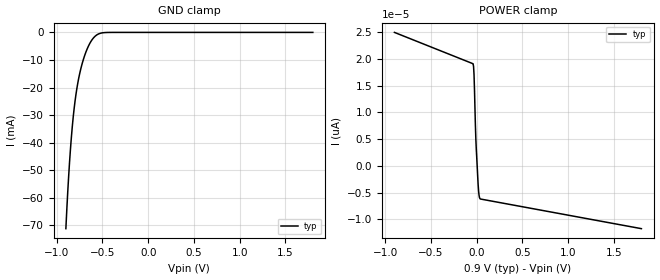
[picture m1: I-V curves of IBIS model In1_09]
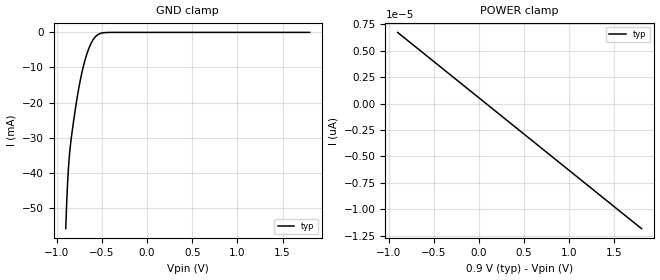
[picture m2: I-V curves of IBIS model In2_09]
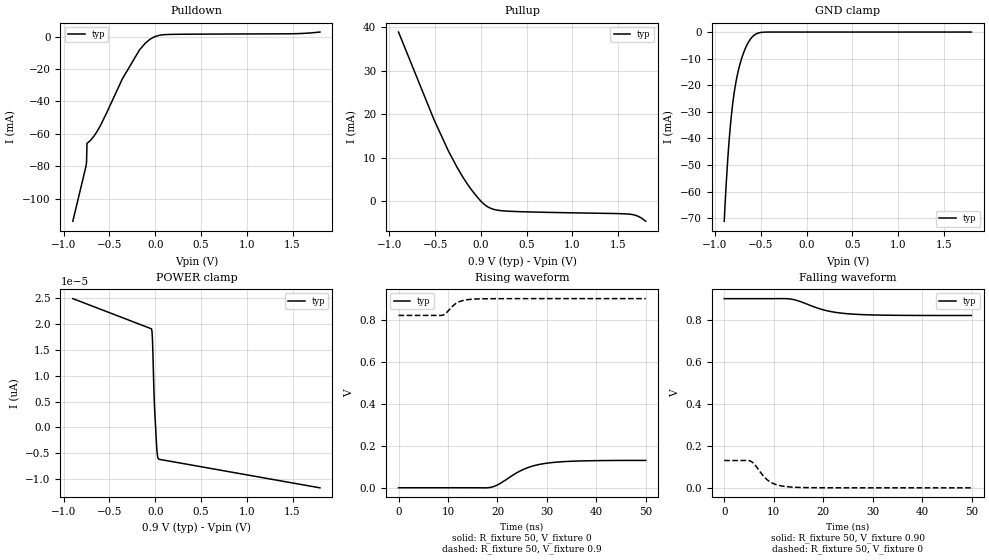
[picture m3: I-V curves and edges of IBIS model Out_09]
|//////////////////////////////////////////////////////////////////////////////
|//////////////////////////////////////////////////////////////////////////////
|   @@@@@@@   @@@@@@@   @@@@@@@   @@@@@@@   @@@@@@@   @@@@@@   @@
|   @@@@@@@@@   @@@@@@@@@   @@@@@@@@@   @@@@@@@@@   @@@@@@@@@ @@@@@@@@  @
|   @@@   @@@ @@@   @@@ @@@   @@@   @@@ @@@   @@@@   @@@  @
|   @@   @@ @@   @@ @@@@@@@@@@@ @@@@@@@@@@@ @@   @@   @@ @@
|   @@@   @@@ @@   @@   @@@ @@@   @@   @@   @@ @@
|   @@@@@@@@@  @@   @@  @@@@@@@@@   @@@@@@@@@  @@   @@   @@ @@
|   @@@@@@@   @@   @@   @@@@@@@   @@@@@@@   @@   @@   @@ @@
|   IBIS Model of NL3V2T244
|   2-Bit Dual-Supply Level Translator
|   Package Type: UDFN8, CASE 517AJ
|   Micro8, CASE 846A-02
|   The model is covering the following Vccs:
|   0.9V, 1.2V, 1.5V, 1.8V, 2.5V, 3.3V
|//////////////////////////////////////////////////////////////////////////////
|//////////////////////////////////////////////////////////////////////////////
[IBIS Ver]   3.2
|   7.2 compatible
|//////////////////////////////////////////////////////////////////////////////
[Comment Char] |_char
|//////////////////////////////////////////////////////////////////////////////
[File Name]   nl3v2t244_va_r0.ibs
|//////////////////////////////////////////////////////////////////////////////
[File Rev]   0.0
|   0.0 - Feb 19, 2025 - File created
|//////////////////////////////////////////////////////////////////////////////
[Date]   February 19, 2025
|//////////////////////////////////////////////////////////////////////////////
[Source]   From lab measurements and simulations at onsemi
|//////////////////////////////////////////////////////////////////////////////
[Notes]   - The currents greater than +/- 100 mA are extrapolated
|//////////////////////////////////////////////////////////////////////////////
[Disclaimer]
   - onsemi Corporation hereby grants
   the user of this IBIS model a license to use this model
   under the following terms. This license is nonexclusive
   and nontransferable. Before using this IBIS model.
   After reading the terms and conditions of this license,
   the user either must accept these terms,
   or the IBIS model should be returned to onsemi within 30 days.
   - The user is hereby granted a license to use the IBIS model.
   This shall not be construed as a right to sell,
   or otherwise profit either by leasing or renting this software.
   - The user may modify the IBIS model to suit his specific
   applications but rights to derivative works and such
   modifications shall belong to onsemi.
   - This IBIS model is provided on an "as is" basis.
   onsemi makes absolutely no warranty with respect
   to the information contained herein.
   By use of this IBIS model, the user assumes full risk as to the
   quality and suitablility of the model to his particular use,
   and by using this model assumes the entire risk.
   Under all circumstances the user shall not hold
   onsemi liable in any way for the results obtained.
   onsemi reserves the right to make to improve
   the model for reliability, function, or design.
   onsemi does not convey any license under patent
   rights or any other intellectual property rights,
   including those of third parties.
   - onsemi is not obligated to provide maintenance
   or support for the licensed IBIS model.
   - Cont onsemi at ATTN:LOGIC APPLICATIONS/IBIS MODEL.
   5701 N Pima Rd, Scottsdale, AZ 85250
|//////////////////////////////////////////////////////////////////////////////
[Copyright]   (c) 2025 onsemi Corp.
|//////////////////////////////////////////////////////////////////////////////
|//////////////////////////////////////////////////////////////////////////////
[Component]   NL3V2T244DMR2G
|//////////////////////////////////////////////////////////////////////////////
[Manufacturer]  onsemi
|   Data Sheet: NL3V2T244/D, Rev. P1,  October, 2024
|//////////////////////////////////////////////////////////////////////////////
[Package]
|   Micro8
| CASE 846A-02
|  DM SUFFIX
| variable   typ   min   max
R_pkg   0.1829   0.0061   0.2446
L_pkg   2.8385nH   1.565nH   3.89485nH
C_pkg   0.4567pF   0.38386pF   0.53234pF
|//////////////////////////////////////////////////////////////////////////////
[Pin] signal_name   model_name   R_pin   L_pin   C_pin
1   VCCA   POWER   0.1862   2.8664nH   0.4560pF
2   A1   In1   0.2446   3.8949nH   0.5323pF
3   A2   In1   0.2357   3.2912nH   0.4714pF
4   OE   In2   0.1867   2.8664nH   0.4559pF
5   GND   GND   0.1866   1.5684nH   0.3839pF
6   B2   Out   0.2341   3.8112nH   0.5277pF
7   B1   Out   0.0061   1.5650nH   0.3853pF
8   VCCB   POWER   0.1830   2.8445nH   0.4412pF
|//////////////////////////////////////////////////////////////////////////////
|//////////////////////////////////////////////////////////////////////////////
[Component]   NL3V2T244DMR2G-Q
|//////////////////////////////////////////////////////////////////////////////
[Manufacturer]  onsemi
|   Data Sheet: NL3V2T244/D, Rev. P1,  October, 2024
|//////////////////////////////////////////////////////////////////////////////
[Package]
R_pkg   0.1829   0.0061   0.2446
L_pkg   2.8385nH   1.565nH   3.89485nH
C_pkg   0.4567pF   0.38386pF   0.53234pF
|//////////////////////////////////////////////////////////////////////////////
[Pin] signal_name   model_name   R_pin   L_pin   C_pin
1   VCCA   POWER   0.1862   2.8664nH   0.4560pF
2   A1   In1   0.2446   3.8949nH   0.5323pF
3   A2   In1   0.2357   3.2912nH   0.4714pF
4   OE   In2   0.1867   2.8664nH   0.4559pF
5   GND   GND   0.1866   1.5684nH   0.3839pF
6   B2   Out   0.2341   3.8112nH   0.5277pF
7   B1   Out   0.0061   1.5650nH   0.3853pF
8   VCCB   POWER   0.1830   2.8445nH   0.4412pF
|//////////////////////////////////////////////////////////////////////////////
|//////////////////////////////////////////////////////////////////////////////
[Component]   NL3V2T244MUTAG
|//////////////////////////////////////////////////////////////////////////////
[Manufacturer]  onsemi
|   Data Sheet: NL3V2T244/D, Rev. P1,  October, 2024
|//////////////////////////////////////////////////////////////////////////////
[Package]
|   UDFN_8
| CASE 517AJ
|  MU SUFFIX
| variable   typ   min   max
R_pkg   0.0451   0.0011   0.0571
L_pkg   0.3714nH   0.01454nH  0.4787nH
C_pkg   0.1048pF   0.07664pF  0.1133pF
|//////////////////////////////////////////////////////////////////////////////
[Pin] signal_name   model_name   R_pin   L_pin   C_pin
1   VCCA   POWER   0.0486   0.3921nH  0.1052pF
2   A1   In1   0.0469   0.3815nH  0.1078pF
3   A2   In1   0.0570   0.4787nH  0.1129pF
4   OE   In2   0.0544   0.4523nH  0.1100pF
5   GND   GND   0.0011   0.0145nH  0.0766pF
6   B2   Out   0.0571   0.4787nH  0.1133pF
7   B1   Out   0.0470   0.3814nH  0.1077pF
8   VCCB   POWER   0.0486   0.3922nH  0.1052pF
|//////////////////////////////////////////////////////////////////////////////
|//////////////////////////////////////////////////////////////////////////////
[Model Selector]   In1
In1_09   Vcc = 0.90
In1_12   Vcc = 1.20
In1_15   Vcc = 1.50
In1_18   Vcc = 1.80
In1_25   Vcc = 2.50
In1_33   Vcc = 3.30
|//////////////////////////////////////////////////////////////////////////////
[Model Selector]   In2
In2_09   Vcc = 0.90
In2_12   Vcc = 1.20
In2_15   Vcc = 1.50
In2_18   Vcc = 1.80
In2_25   Vcc = 2.50
In2_33   Vcc = 3.30
|//////////////////////////////////////////////////////////////////////////////
[Model Selector]   Out
Out_09   Vcc = 0.90
Out_12   Vcc = 1.20
Out_15   Vcc = 1.50
Out_18   Vcc = 1.80
Out_25   Vcc = 2.50
Out_33   Vcc = 3.30
| Models and submodels in the file (18): In1_09 (Input), In2_09 (Input), Out_09 (3-state), In1_12 (Input), In2_12 (Input), Out_12 (3-state), In1_15 (Input), In2_15 (Input), Out_15 (3-state), In1_18 (Input), In2_18 (Input), Out_18 (3-state), In1_25 (Input), In2_25 (Input), Out_25 (3-state), In1_33 (Input), In2_33 (Input), Out_33 (3-state)
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|//////////////////////////////////////////////////////////////////////////////
|//////////////////////////////////////////////////////////////////////////////
[Model]  In1_09
Model_type Input
Vinh =  0.81
Vinl =  0.09
|  variable   typ   min   max
C_comp   6.2pF   6.2pF   6.2pF
|//////////////////////////////////////////////////////////////////////////////
[Temperature Range]   25   125   -40
|//////////////////////////////////////////////////////////////////////////////
[Voltage Range]   0.90V   NA   NA
|//////////////////////////////////////////////////////////////////////////////
[POWER Clamp Reference] 0.90V   NA   NA
|//////////////////////////////////////////////////////////////////////////////
[GND Clamp Reference]   0V   NA   NA
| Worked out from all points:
|   GND clamp passes 1 mA (typ) near -0.57 V on its own axis
|//////////////////////////////////////////////////////////////////////////////
[GND Clamp]
|   Voltage   I(typ)   I(min)   I(max)
-900mV    -71.17mA   NA         NA
-880mV    -58.1mA    NA         NA
-870mV    -52.38mA   NA         NA
-840mV    -38.09mA   NA         NA
-810mV    -27.71mA   NA         NA
-780mV    -20.38mA   NA         NA
-740mV    -13.65mA   NA         NA
-690mV    -7.952mA   NA         NA
-630mV    -3.503mA   NA         NA
-570mV    -1.104mA   NA         NA
-430mV    -13.71uA   NA         NA
1.8V      -3.229pA   NA         NA
|//////////////////////////////////////////////////////////////////////////////
[POWER Clamp]
|   Voltage   I(typ)   I(min)   I(max)
-900mV    24.95pA    NA         NA
-40mV     19.09pA    NA         NA
-35mV     18.58pA    NA         NA
-30mV     17.13pA    NA         NA
-25mV     14.37pA    NA         NA
-15mV     7.634pA    NA         NA
-10mV     5.037pA    NA         NA
-5mV      3.078pA    NA         NA
15mV      -3.465pA   NA         NA
25mV      -5.478pA   NA         NA
40mV      -6.189pA   NA         NA
1.8V      -11.73pA   NA         NA
|//////////////////////////////////////////////////////////////////////////////
|//////////////////////////////////////////////////////////////////////////////
[Model]  In2_09
Model_type Input
Vinh =  0.81
Vinl =  0.09
|  variable   typ   min   max
C_comp   4.8pF   4.8pF   4.8pF
|//////////////////////////////////////////////////////////////////////////////
[Temperature Range]   25   125   -40
|//////////////////////////////////////////////////////////////////////////////
[Voltage Range]   0.90V   NA   NA
|//////////////////////////////////////////////////////////////////////////////
[POWER Clamp Reference] 0.90V   NA   NA
|//////////////////////////////////////////////////////////////////////////////
[GND Clamp Reference]   0V   NA   NA
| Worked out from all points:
|   GND clamp passes 1 mA (typ) near -0.56 V on its own axis
|//////////////////////////////////////////////////////////////////////////////
[GND Clamp]
|   Voltage   I(typ)   I(min)   I(max)
-900mV    -55.97mA   NA         NA
-890mV    -49.01mA   NA         NA
-880mV    -43.23mA   NA         NA
-860mV    -35.28mA   NA         NA
-830mV    -28.47mA   NA         NA
-780mV    -19.63mA   NA         NA
-730mV    -12.54mA   NA         NA
-680mV    -7.319mA   NA         NA
-620mV    -3.149mA   NA         NA
-560mV    -954.7uA   NA         NA
-420mV    -11.1uA    NA         NA
1.8V      6.738pA    NA         NA
|//////////////////////////////////////////////////////////////////////////////
[POWER Clamp]
|   Voltage   I(typ)   I(min)   I(max)
-900mV    6.738pA    NA         NA
0V        548.1fA    NA         NA
900mV     -5.642pA   NA         NA
1.8V      -11.83pA   NA         NA
|//////////////////////////////////////////////////////////////////////////////
|//////////////////////////////////////////////////////////////////////////////
[Model] Out_09
Model_type 3-state
Polarity Non-Inverting
Enable Active-Low
Vmeas = 0.45
Vref = 0.9
Rref = 2k
Cref = 15pF
|  variable   typ   min   max
C_comp   5.9pF   5.9pF   5.9pF
|//////////////////////////////////////////////////////////////////////////////
[Temperature Range]   25   125   -40
|//////////////////////////////////////////////////////////////////////////////
[Voltage Range]   0.90V   NA   NA
|//////////////////////////////////////////////////////////////////////////////
[Pulldown Reference]   0V   NA   NA
|//////////////////////////////////////////////////////////////////////////////
[Pullup Reference]   0.90V   NA   NA
|//////////////////////////////////////////////////////////////////////////////
[GND Clamp Reference]   0V   NA   NA
|//////////////////////////////////////////////////////////////////////////////
[POWER Clamp Reference] 0.90V   NA   NA
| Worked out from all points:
|   slope of the pulldown table from 0 to 0.135 V, typ, clamps not added: 105 ohm
|   slope of the pullup table from 0 to 0.135 V, typ, clamps not added: 73.3 ohm
|   GND clamp passes 1 mA (typ) near -0.57 V on its own axis
|   falling waveform, R_fixture 50, V_fixture 0.90: 20-80 % time 6.55ns typ, NA min, NA max; typ from 0.9 V to 0.82 V
|   falling waveform, R_fixture 50, V_fixture 0: 20-80 % time 3.06ns typ, NA min, NA max; typ from 0.13 V to 0 V
|   rising waveform, R_fixture 50, V_fixture 0: 20-80 % time 6.32ns typ, NA min, NA max; typ from 0 V to 0.13 V
|   rising waveform, R_fixture 50, V_fixture 0.9: 20-80 % time 2.34ns typ, NA min, NA max; typ from 0.82 V to 0.9 V
|//////////////////////////////////////////////////////////////////////////////
[Pulldown]
|   Voltage   I(typ)   I(min)   I(max)
-900mV    -114mA     NA         NA
-755mV    -79.79mA   NA         NA
-750mV    -77.44mA   NA         NA
-745mV    -65.81mA   NA         NA
-670mV    -61.49mA   NA         NA
-595mV    -54.58mA   NA         NA
-360mV    -26.24mA   NA         NA
-170mV    -8.078mA   NA         NA
-60mV     -1.806mA   NA         NA
20mV      397.5uA    NA         NA
130mV     1.272mA    NA         NA
1.8V      2.798mA    NA         NA
|//////////////////////////////////////////////////////////////////////////////
[Pullup]
|   Voltage   I(typ)   I(min)   I(max)
-900mV    38.91mA    NA         NA
-515mV    18.89mA    NA         NA
-360mV    11.76mA    NA         NA
-260mV    7.771mA    NA         NA
-150mV    4.012mA    NA         NA
-30mV     716.4uA    NA         NA
50mV      -948.5uA   NA         NA
140mV     -1.873mA   NA         NA
280mV     -2.276mA   NA         NA
1.63V     -2.998mA   NA         NA
1.72V     -3.503mA   NA         NA
1.8V      -4.62mA    NA         NA
|//////////////////////////////////////////////////////////////////////////////
[GND Clamp]
|   Voltage   I(typ)   I(min)   I(max)
-900mV    -71.17mA   NA         NA
-880mV    -58.1mA    NA         NA
-870mV    -52.38mA   NA         NA
-840mV    -38.09mA   NA         NA
-810mV    -27.71mA   NA         NA
-780mV    -20.38mA   NA         NA
-740mV    -13.65mA   NA         NA
-690mV    -7.952mA   NA         NA
-630mV    -3.503mA   NA         NA
-570mV    -1.104mA   NA         NA
-430mV    -13.71uA   NA         NA
1.8V      -3.229pA   NA         NA
|//////////////////////////////////////////////////////////////////////////////
[POWER Clamp]
|   Voltage   I(typ)   I(min)   I(max)
-900mV    24.95pA    NA         NA
-40mV     19.09pA    NA         NA
-35mV     18.58pA    NA         NA
-30mV     17.13pA    NA         NA
-25mV     14.37pA    NA         NA
-15mV     7.634pA    NA         NA
-10mV     5.037pA    NA         NA
-5mV      3.078pA    NA         NA
15mV      -3.465pA   NA         NA
25mV      -5.478pA   NA         NA
40mV      -6.189pA   NA         NA
1.8V      -11.73pA   NA         NA
|//////////////////////////////////////////////////////////////////////////////
|//////////////////////////////////////////////////////////////////////////////
[Ramp]
|  variable   typ   min   max
dV/dt_r   7.800E-02/6.300E-09  7.800E-02/6.300E-09  7.800E-02/6.300E-09
dV/dt_f   4.800E-02/6.300E-09  4.800E-02/6.300E-09  4.800E-02/6.300E-09
R_load = 50
|//////////////////////////////////////////////////////////////////////////////
[Falling Waveform]
R_fixture = 50
V_fixture = 0.90
C_fixture = 0p
|   time   V(typ)   V(min)   V(max)
0s        900mV      NA         NA
12ns      900.2mV    NA         NA
13.2ns    898.8mV    NA         NA
15ns      889.2mV    NA         NA
18.6ns    857.2mV    NA         NA
20.4ns    844.6mV    NA         NA
22.8ns    833.8mV    NA         NA
25.8ns    826.8mV    NA         NA
33.6ns    821.1mV    NA         NA
49.95ns   820mV      NA         NA
|//////////////////////////////////////////////////////////////////////////////
[Falling Waveform]
R_fixture = 50
V_fixture = 0
C_fixture = 0p
|   time   V(typ)   V(min)   V(max)
0s        130mV      NA         NA
4.65ns    130.2mV    NA         NA
5.25ns    127.7mV    NA         NA
6ns       114.7mV    NA         NA
7.8ns     59.55mV    NA         NA
9ns       32.71mV    NA         NA
10.5ns    15.27mV    NA         NA
12.6ns    5.671mV    NA         NA
18.55ns   558.6uV    NA         NA
49.95ns   0V         NA         NA
|//////////////////////////////////////////////////////////////////////////////
[Rising Waveform]
R_fixture = 50
V_fixture = 0
C_fixture = 0p
|   time   V(typ)   V(min)   V(max)
0s        0V         NA         NA
18.3ns    680.3uV    NA         NA
20.1ns    14.65mV    NA         NA
23.7ns    68.44mV    NA         NA
25.2ns    86.8mV     NA         NA
27ns      102.4mV    NA         NA
29.1ns    113.6mV    NA         NA
32.1ns    122.1mV    NA         NA
36ns      126.9mV    NA         NA
49.95ns   130mV      NA         NA
|//////////////////////////////////////////////////////////////////////////////
[Rising Waveform]
R_fixture = 50
V_fixture = 0.9
C_fixture = 0p
|   time   V(typ)   V(min)   V(max)
0s        820mV      NA         NA
8.85ns    820.8mV    NA         NA
9.15ns    823.3mV    NA         NA
9.45ns    828mV      NA         NA
11.1ns    867.7mV    NA         NA
12ns      882.2mV    NA         NA
13.2ns    891.9mV    NA         NA
15ns      897.3mV    NA         NA
20.15ns   899.8mV    NA         NA
49.95ns   900mV      NA         NA
